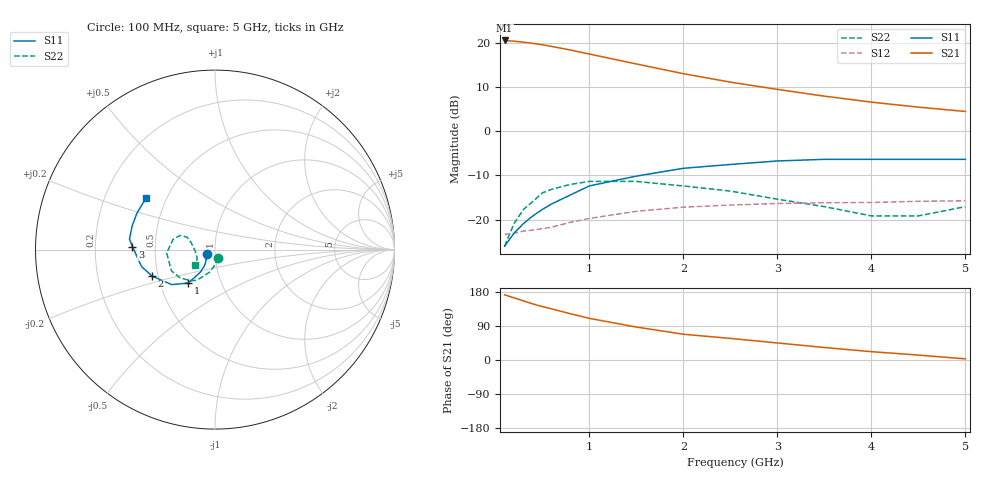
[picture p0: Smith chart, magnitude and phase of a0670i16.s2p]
!  MSA-0670 S AND NOISE PARAMETERS
!  Id=16mA  LAST UPDATED 07-22-92
# ghz s ma r 50
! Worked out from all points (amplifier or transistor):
!   16 points, 100 MHz to 5 GHz, reference 50 ohm
!   highest |S21| = 20.5 dB at 100 MHz (marker M1)
!   |S21| within 3 dB of that: start of sweep to 985 MHz
!   unconditionally stable (mu >= 1): start of sweep to 419.9 MHz; 2.448 GHz to end of sweep
!   at 300 MHz: K = 1.02, MAG = 20.6 dB, |S12| = -22.6 dB
!   at 1.5 GHz: K = 0.91, MSG = 16.7 dB, |S12| = -18.1 dB
!   at 5 GHz: K = 1.45, MAG = 6.1 dB, |S12| = -15.8 dB
!   lowest NFmin = 2.70 dB at 100 MHz
!   S11 on the Smith chart (normalised r, x): 100 MHz: 0.92, -0.05; 1 GHz: 0.69, -0.27; 2 GHz: 0.46, -0.16; 3 GHz: 0.37, +0.02; 5 GHz: 0.39, +0.29
0.1  0.05 -147.0  10.62 172.0  0.068 4.0  0.05 -69.0
0.2  0.07 -134.0  10.41 164.0  0.07 8.0  0.09 -92.0
0.3  0.09 -126.0  10.16 156.0  0.074 12.0  0.13 -104.0
0.4  0.11 -123.0  9.85 148.0  0.076 14.0  0.16 -113.0
0.5  0.13 -123.0  9.5 141.0  0.079 16.0  0.2 -121.0
0.6  0.15 -123.0  9.09 135.0  0.082 18.0  0.22 -128.0
0.8  0.19 -126.0  8.28 122.0  0.093 22.0  0.25 -141.0
1  0.24 -129.0  7.46 110.0  0.103 22.0  0.27 -154.0
1.5  0.31 -141.0  5.76 87.0  0.124 23.0  0.27 -176.0
2  0.38 -157.0  4.47 68.0  0.138 19.0  0.24 166.0
2.5  0.42 -167.0  3.59 57.0  0.146 20.0  0.21 158.0
3  0.46 178.0  2.97 45.0  0.152 16.0  0.17 156.0
3.5  0.48 173.0  2.49 33.0  0.155 11.0  0.14 163.0
4  0.48 164.0  2.13 22.0  0.156 9.0  0.11 -175.0
4.5  0.48 155.0  1.87 13.0  0.161 5.0  0.11 -154.0
5  0.48 143.0  1.67 3.0  0.163 3.0  0.14 -141.0
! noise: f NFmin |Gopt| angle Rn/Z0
0.1  2.7  0.11  6  0.4
0.5  2.8  0.11  29  0.39
1  3  0.11  62  0.38
2  3.3  0.13  125  0.35
